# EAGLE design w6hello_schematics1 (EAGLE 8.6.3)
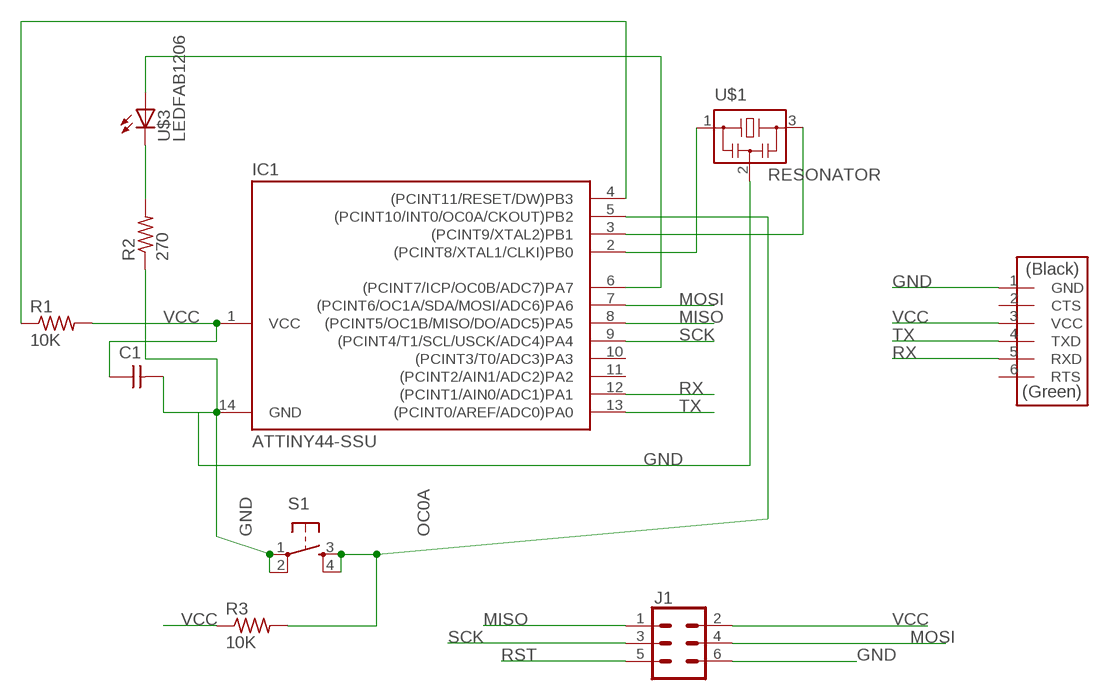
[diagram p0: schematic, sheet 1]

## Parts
C1  CAP-UNPOLARIZEDFAB  [C1206FAB]
IC1  ATTINY44-SSU  [SOIC14]
J1  CONN_03X2SMT  [2X3_SMT_POSTS]
R1  10K  RES-US1206FAB  [R1206FAB]
R2  270  RES-US1206FAB  [R1206FAB]
R3  10K  RES-US1206FAB  [R1206FAB]
S1  6MM_SWITCH6MM_SWITCH  [6MM_SWITCH]
U$1  RESONATOR  [EFOBM]
U$2  FTDI-SMD-HEADER  [1X06SMD]
U$3  LEDFAB1206  [LED1206FAB]

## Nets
GND: C1.2 IC1.14(GND) J1.6 R2.1 S1.1(P) S1.2(P1) U$1.2 U$2.1(GND)
MISO: IC1.8((PCINT5/OC1B/MISO/DO/ADC5)PA5) J1.1
MOSI: IC1.7((PCINT6/OC1A/SDA/MOSI/ADC6)PA6) J1.4
N$1: IC1.2((PCINT8/XTAL1/CLKI)PB0) U$1.1
N$2: IC1.3((PCINT9/XTAL2)PB1) U$1.3
N$3: IC1.6((PCINT7/ICP/OC0B/ADC7)PA7) U$3.1(A)
N$4: R2.2 U$3.2(C)
OC0A: IC1.5((PCINT10/INT0/OC0A/CKOUT)PB2) R3.2 S1.3(S) S1.4(S1)
RST: IC1.4((PCINT11/RESET/DW)PB3) J1.5 R1.1
RX: IC1.12((PCINT1/AIN0/ADC1)PA1) U$2.5(RXD)
SCK: IC1.9((PCINT4/T1/SCL/USCK/ADC4)PA4) J1.3
TX: IC1.13((PCINT0/AREF/ADC0)PA0) U$2.4(TXD)
VCC: C1.1 IC1.1(VCC) J1.2 R1.2 R3.1 U$2.3(VCC)
Unconnected: IC1.10((PCINT3/T0/ADC3)PA3) IC1.11((PCINT2/AIN1/ADC2)PA2) U$2.2(CTS) U$2.6(RTS)

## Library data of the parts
C1 = fab:CAP-UNPOLARIZED
IC1 = fab:ATTINY44
J1 = fab:CONN_03X2: Multi connection point. Often used as Generic Header-pin footprint for 0.1 inch spaced/style header connections You can populate with any combo of single row headers, but if you'd like an exact match, check these: Header - 2x3 (Male, 0.1") (PRT-12807) Header - 2x3 (Female, 0.1") (PRT-13010) 2x3 Pin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; PROD_ID: CONN-11415
R1-R3 = fab:RES-US: Resistor (US Symbol)
S1 = fab:6MM_SWITCH: OMRON SWITCH
U$1 = fab:RESONATOR
U$2 = fab:FTDI-SMD-HEADER
U$3 = fab:LED: LED

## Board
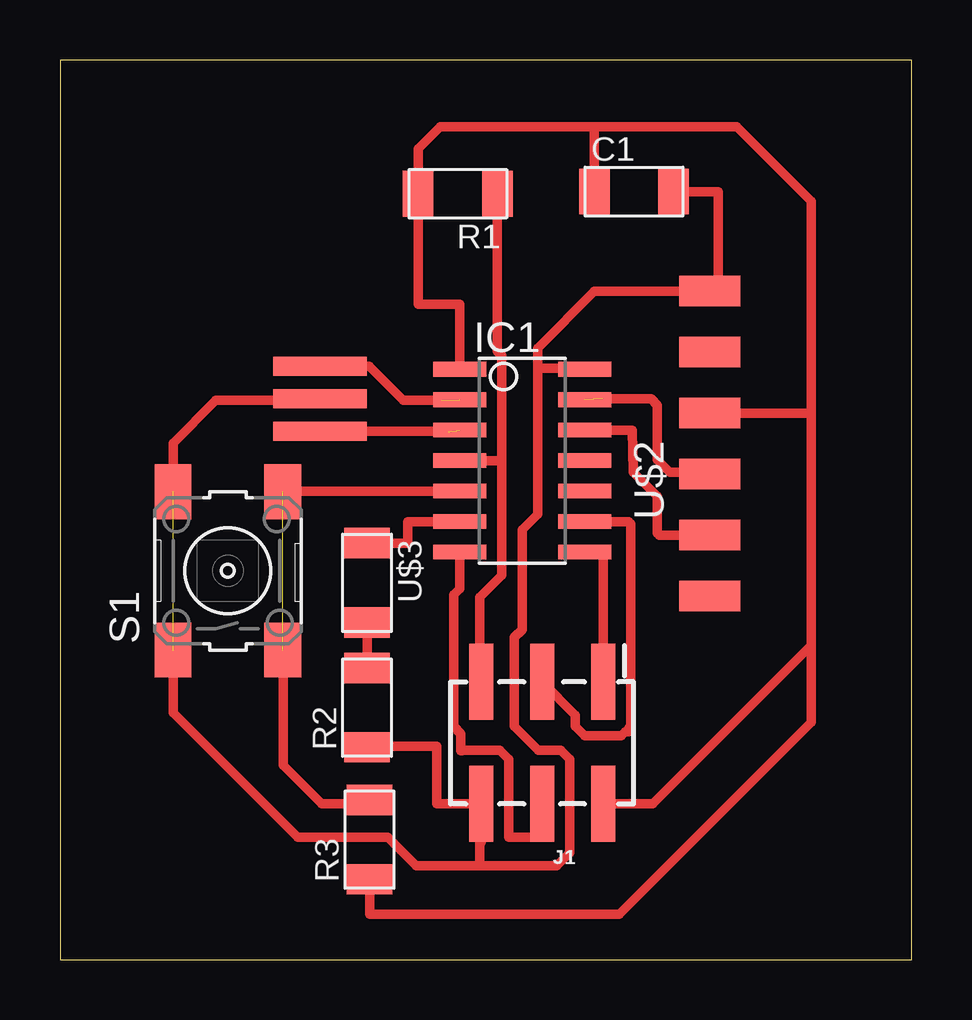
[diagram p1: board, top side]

Size 35.49 x 37.49 mm. Coordinates in mm from the lower left corner, seen from the top.
Outline: 0,0 35.49,0 35.49,37.49 0,37.49 0,0
Copper layers (1*16): Top 0.035mm / dielectric 1.5mm / Bottom 0.035mm
Design rules "default *": minimum track width 6mil, minimum drill 0.35mm, track to track 0.45mm, track to pad 0.45mm, pad to pad 0.45mm, via to via 0.45mm, smd to smd 0.45mm, copper to edge 40mil, drill to drill 6mil, minimum pad ring 10mil, minimum via ring 8mil, stop-mask expansion 4mil, vias tented up to drill 0mil, thermal gap 10mil

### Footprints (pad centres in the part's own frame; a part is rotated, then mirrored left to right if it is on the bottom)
C1206FAB = smd 1.27 x 1.905: 1 -1.651,0; 2 1.651,0
SOIC14 = smd 0.61 x 2.21: 1 -3.81,-2.603; 2 -2.54,-2.603; 3 -1.27,-2.603; 4 0,-2.603; 5 1.27,-2.603; 6 2.54,-2.603; 7 3.81,-2.603; 8 3.81,2.603; 9 2.54,2.603; 10 1.27,2.603; 11 0,2.603; 12 -1.27,2.603; 13 -2.54,2.603; 14 -3.81,2.603
2X3_SMT_POSTS = smd 1 x 3.17: 1 -2.54,-2.54; 2 -2.54,2.54; 3 0,-2.54; 4 0,2.54; 5 2.54,-2.54; 6 2.54,2.54
R1206FAB = smd 1.27 x 1.905: 1 -1.651,0; 2 1.651,0
6MM_SWITCH = smd 2.286 x 1.524: 1 -3.302,2.286; 2 3.302,2.286; 3 -3.302,-2.286; 4 3.302,-2.286
EFOBM = smd 0.8 x 3.9: 1 -1.35,0; 2 0,0; 3 1.35,0
1X06SMD = smd 2.54 x 1.27: 1 0,6.35; 2 0,3.81; 3 0,1.27; 4 0,-1.27; 5 0,-3.81; 6 0,-6.35
LED1206FAB = smd 1.27 x 1.905: 1 -1.651,0; 2 1.651,0

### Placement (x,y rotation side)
C1  23.92,32.01 0 top
IC1  19.26,20.8 270 top
J1  20.09,9.04 180 top
R1  16.58,31.92 180 top
R2  12.8,10.51 90 top
R3  12.9,5.01 90 top
S1  7,16.21 90 top
U$1  10.83,23.38 270 top
U$2  27.08,21.51 0 top
U$3  12.8,15.71 270 top

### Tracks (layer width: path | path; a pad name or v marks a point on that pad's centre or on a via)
GND  (1 unrouted)
  Top 0.4: 17.5,3.91 20.7,3.91 21.24,4.45 21.24,8.35 20.86,8.73 19.93,8.73 18.94,9.72 18.94,13.43 19.26,13.75 19.26,17.91 19.9,18.55 19.9,24.64 | J1.6 17.5,6.5 17.5,4.91 | 17.5,3.91 17.5,4.91 | J1.6 15.7,6.51 15.7,8.91 12.8,8.91 R2.1 | 17.5,3.91 14.84,3.91 13.65,5.11 9.9,5.11 4.71,10.29 S1.1 | 22.4,24.61 IC1.14 | IC1.14 21.4,24.61 | 17.5,4.91 17.55,4.91 J1.6 | U$1.2 10.76,23.31 6.5,23.31 4.71,21.52 S1.2 | C1.2 27.43,32 27.43,28.21 U$2.1 22.27,27.86 19.9,25.48 19.9,24.64 | IC1.14 21.83,24.64 19.9,24.64
MISO
  Top 0.4: IC1.8 22.63,16.99 J1.1
MOSI
  Top 0.4: IC1.7 16.65,15.46 16.4,15.21 16.4,9.72 16.7,9.42 16.7,8.71 16.75,8.71 16.78,8.73 18.32,8.73 18.7,8.35 18.7,5.11 20.1,5.11 J1.4
N$1  (1 unrouted)
  Top 0.4: U$1.1 12.88,24.73 14.3,23.31 15.9,23.31
N$2  (1 unrouted)
  Top 0.4: U$1.3 16.18,22.03 16.2,22.01
N$3
  Top 0.4: U$3.1 14.5,17.36 14.5,18.26 IC1.6
N$4
  Top 0.4: U$3.2 R2.2
OC0A  (1 unrouted)
  Top 0.4: R3.2 12.75,6.51 10.9,6.51 9.3,8.11 9.3,12.89 S1.3 | IC1.5 9.3,19.53 S1.4
RST
  Top 0.4: R1.1 18.23,25.36 18.41,25.18 18.41,20.8 | J1.5 17.5,11.58 17.5,15.11 18.41,16.02 18.41,20.71 18.41,20.8 | 18.41,20.8 IC1.4
RX
  Top 0.4: U$2.5 24.98,17.7 24.89,17.78 24.89,19.3 23.88,20.32 23.84,22.07 IC1.12
SCK
  Top 0.4: IC1.9 23.7,18.26 23.78,18.18 23.78,9.72 23.7,9.64 23.7,9.51 23.56,9.51 23.39,9.34 21.86,9.34 21.48,9.72 21.48,10.19 J1.3
TX  (1 unrouted)
  Top 0.4: U$2.4 26.99,20.32 25.4,20.32 24.89,20.83 24.89,23.11 24.64,23.37 22.61,23.37
VCC
  Top 0.4: 31.3,22.71 31.3,13.1 | R3.1 12.9,1.91 23.3,1.91 31.3,9.91 31.3,13.1 | J1.2 24.7,6.5 31.3,13.1 | 22.27,34.71 28.19,34.71 31.3,31.6 31.3,22.71 | IC1.1 16.65,27.31 14.93,27.31 R1.2 14.93,33.78 15.85,34.71 22.27,34.71 | C1.1 22.27,34.71 | U$2.3 31.23,22.78 31.3,22.71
